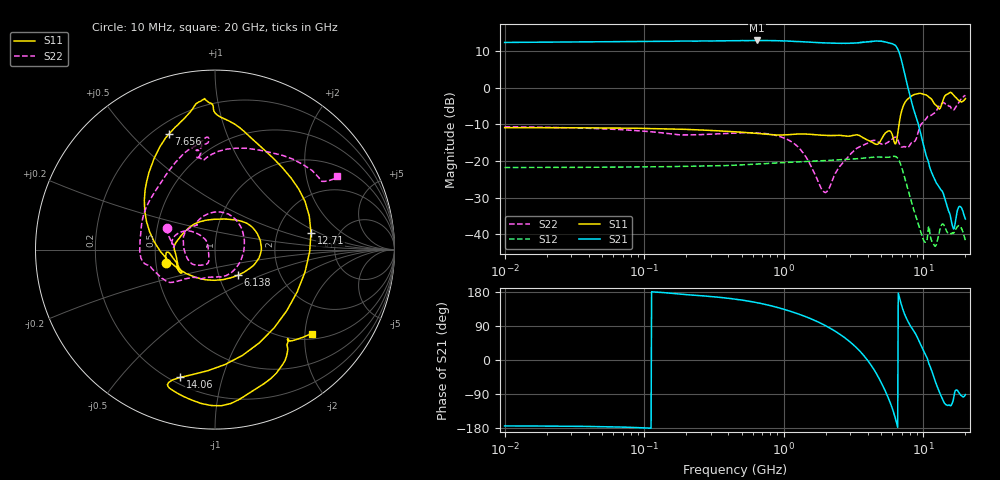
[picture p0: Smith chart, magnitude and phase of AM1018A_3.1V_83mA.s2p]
!	"Atlanta Micro, Inc."
!	Email:	infoatlantamicro.com		Phone:	470-253-7640
!	Model Number:	AM1018A		Date:	17-Mar
!	Filename:	AM1018A_3.1V_83mA.s2p	Version:1.0
!	Description:	2-port S-parameter data for AM1018A amplifier
!	Frequency Range:	10 MHz to 20 GHz
!	Port Configuration:	"Port 1: Input (pin 3), Port 2: Output (pin 10)"
!	"S2P File: Measurements: S11, S21, S12, S22:"
#	GHz	S	dB	R	50
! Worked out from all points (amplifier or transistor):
!   827 points, 10 MHz to 20 GHz, reference 50 ohm
!   highest |S21| = 13.0 dB at 642.7 MHz (marker M1)
!   |S21| within 3 dB of that: start of sweep to 6.665 GHz
!   unconditionally stable (mu >= 1): start of sweep to end of sweep
!   at 35.3 MHz: K = 1.47, MAG = 13.1 dB, |S12| = -21.7 dB
!   at 448.8 MHz: K = 1.39, MAG = 13.3 dB, |S12| = -21.1 dB
!   at 20 GHz: K = 689.73, MAG = -28.5 dB, |S12| = -41.7 dB
!   S11 on the Smith chart (normalised r, x): 10 MHz: 0.56, -0.09; 6.138 GHz: 1.24, -0.37; 7.656 GHz: 0.26, +0.65; 12.71 GHz: 3.13, +0.83; 14.06 GHz: 0.24, -0.74; 20 GHz: 1.12, -2.16
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0.01  -10.87 -164.3  12.44 -174.0  -21.78 6.4  -10.62 156.1
0.0356  -10.92 -165.6  12.55 -175.1  -21.74 6.0  -10.98 159.5
0.126  -11.13 -171.8  12.72 178.9  -21.59 2.8  -12.19 170.0
0.44875  -11.99 -174.6  12.93 160.6  -21.14 -5.5  -12.34 172.9
0.64269  -12.45 -168.8  12.98 151.3  -20.85 -9.5  -12.32 165.7
1.0375  -12.84 -158.0  12.86 132.1  -20.40 -19.6  -13.94 149.2
1.5996  -12.74 -145.5  12.49 107.3  -20.04 -34.9  -22.06 133.7
2.1478  -13.02 -147.8  12.28 83.9  -19.80 -50.8  -26.82 -139.4
2.7542  -13.13 -163.0  12.19 57.8  -19.59 -69.0  -19.76 -125.0
3.342  -12.83 175.5  12.31 31.3  -19.37 -87.7  -16.49 -147.5
3.9811  -14.26 145.8  12.60 -0.6  -19.08 -110.0  -15.11 173.8
4.6989  -15.42 87.9  12.81 -41.6  -18.90 -137.4  -14.68 138.3
5.2  -12.95 42.0  12.64 -73.0  -18.98 -157.4  -15.42 125.5
5.6494  -11.79 7.7  12.33 -102.8  -18.95 -175.6  -14.67 122.3
6.1376  -14.32 -47.8  11.87 -139.8  -18.72 160.3  -13.64 93.2
6.4863  -13.60 -140.3  10.94 -171.7  -19.05 137.0  -13.84 54.6
6.8549  -7.67 157.4  8.55 154.4  -20.79 111.0  -15.87 -2.7
7.656  -3.18 111.8  0.92 105.7  -27.11 74.2  -16.30 -88.2
10.864  -2.40 89.8  -20.22 -5.3  -38.22 -56.7  -7.63 -173.6
12.706  -5.31 10.0  -26.61 -74.7  -41.06 -76.8  -5.50 115.0
14.06  -2.64 -105.2  -29.51 -111.9  -37.59 -104.0  -4.05 93.6
20  -2.91 -41.2  -35.88 -91.2  -41.74 -94.8  -2.01 31.0
